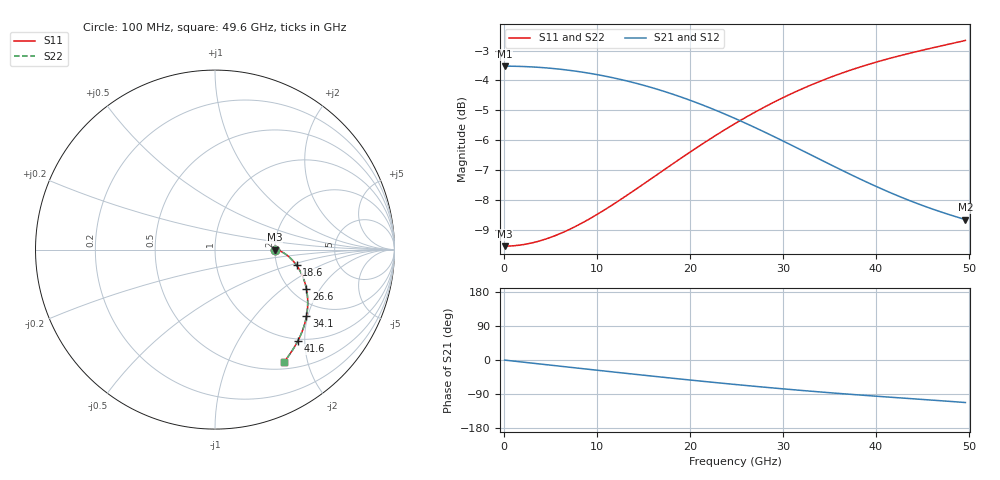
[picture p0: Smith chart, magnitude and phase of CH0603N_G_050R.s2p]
# GHz S RI R 50
! S-Parameters data
! Freq  reS11  imS11  reS21  imS21  reS12  imS12  reS22  imS22
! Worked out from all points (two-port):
!   100 points, 100 MHz to 49.6 GHz, reference 50 ohm
!   highest |S21| = -3.52 dB at 100 MHz (marker M1); lowest = -8.7 dB at 49.6 GHz (marker M2)
!   |S21| within 3 dB of the highest: start of sweep to 33.22 GHz
!   lowest |S11| = -9.5 dB at 100 MHz (marker M3), VSWR 2.00, Z = 100 - j3.44e-06 ohm
!   |S11| at or under -10 dB: nowhere
!   |S22| runs from -9.5 to -2.7 dB; largest |S21 - S12| = 0
!   S11 on the Smith chart (normalised r, x): 100 MHz: 2.00, -0.00; 18.6 GHz: 2.57, -0.57; 26.6 GHz: 2.40, -1.51; 34.1 GHz: 1.60, -1.96; 41.6 GHz: 0.95, -1.85; 49.6 GHz: 0.59, -1.62
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0.1  0.3333 -1.53e-08  0.6667 -0.00314  0.6667 -0.00314  0.3333 -1.53e-08
2.1  0.3354 -0.000141  0.6625 -0.0658  0.6625 -0.0658  0.3354 -0.000141
4.1  0.341 -0.00105  0.6508 -0.1272  0.6508 -0.1272  0.341 -0.00105
6.1  0.35 -0.00343  0.6318 -0.1865  0.6318 -0.1865  0.35 -0.00343
8.6  0.3656 -0.00952  0.5986 -0.2558  0.5986 -0.2558  0.3656 -0.00952
10.6  0.3809 -0.0176  0.5651 -0.3064  0.5651 -0.3064  0.3809 -0.0176
12.6  0.3982 -0.0291  0.5264 -0.3518  0.5264 -0.3518  0.3982 -0.0291
14.6  0.4167 -0.0444  0.4833 -0.3913  0.4833 -0.3913  0.4167 -0.0444
16.6  0.4357 -0.0638  0.437 -0.4245  0.437 -0.4245  0.4357 -0.0638
18.6  0.4543 -0.0873  0.3884 -0.4511  0.3884 -0.4511  0.4543 -0.0873
20.1  0.4675 -0.1076  0.3512 -0.4666  0.3512 -0.4666  0.4675 -0.1076
21.6  0.4797 -0.1301  0.3138 -0.4785  0.3138 -0.4785  0.4797 -0.1301
23.1  0.4906 -0.1546  0.2767 -0.4867  0.2767 -0.4867  0.4906 -0.1546
25.1  0.5025 -0.19  0.2284 -0.4925  0.2284 -0.4925  0.5025 -0.19
26.6  0.5092 -0.2183  0.1935 -0.4932  0.1935 -0.4932  0.5092 -0.2183
30.1  0.5165 -0.2881  0.1181 -0.4848  0.1181 -0.4848  0.5165 -0.2881
33.1  0.5129 -0.3496  0.0615 -0.4689  0.0615 -0.4689  0.5129 -0.3496
34.1  0.5098 -0.37  0.0443 -0.4624  0.0443 -0.4624  0.5098 -0.37
37.6  0.4917 -0.439  -0.00894 -0.4367  -0.00894 -0.4367  0.4917 -0.439
41.6  0.4605 -0.5109  -0.059 -0.4049  -0.059 -0.4049  0.4605 -0.5109
45.6  0.423 -0.5734  -0.1011 -0.3734  -0.1011 -0.3734  0.423 -0.5734
49.6  0.3842 -0.6278  -0.1396 -0.3419  -0.1396 -0.3419  0.3842 -0.6278
